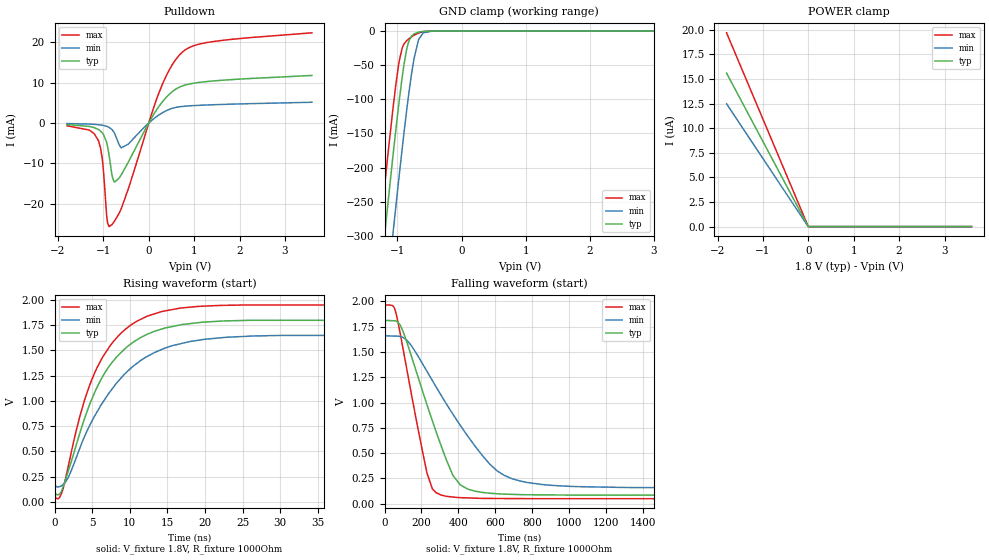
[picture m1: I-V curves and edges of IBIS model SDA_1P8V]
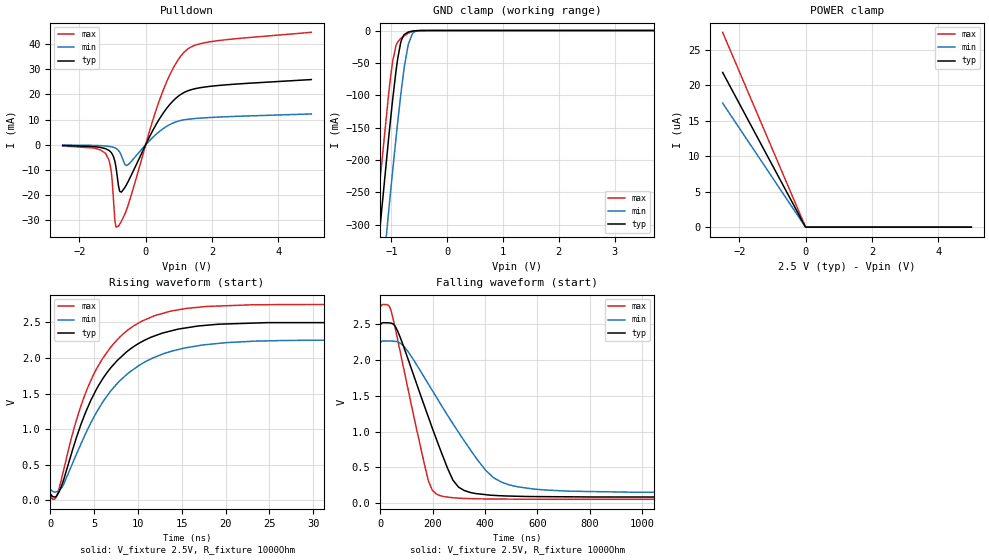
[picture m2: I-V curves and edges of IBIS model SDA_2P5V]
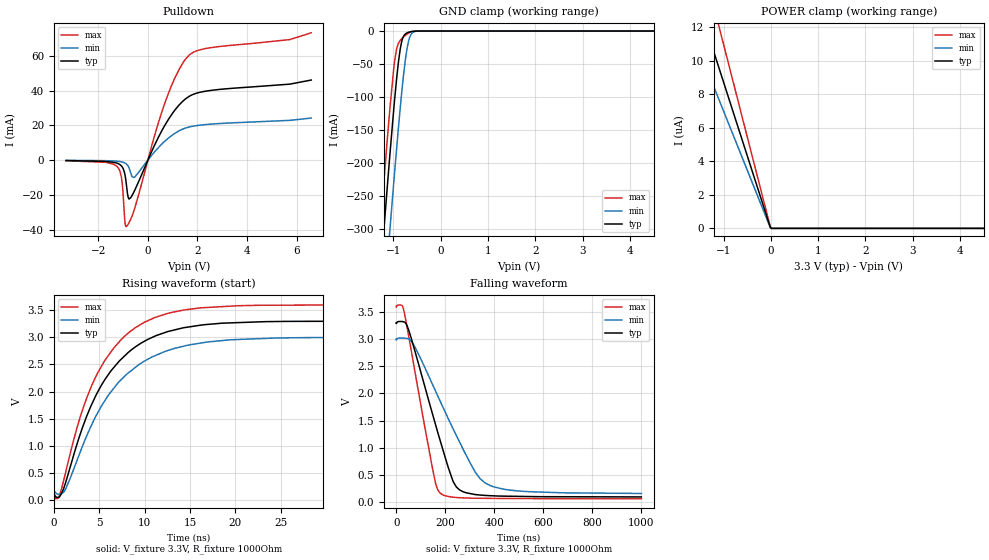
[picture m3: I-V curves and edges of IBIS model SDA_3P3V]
| Texas Instruments Incorporated
| LOW VOLTAGE 8-BIT I2C AND SMBus LOW-POWER I/O EXPANDER
| WITH INTERRUPT OUTPUT, RESET, AND CONFIGURATION REGISTERS
| Marketing part#   Voltage Range   Package-type   #pins/pkg drawing
| TCA9534PW   1.65V - 5.5V   TSSOP   16-pin PW
| TCA9534APW   1.65V - 5.5V   TSSOP   16-pin PW
[IBIS Ver]   4.1
[File name]   tca9534.ibs
[File Rev]   1.0
[Date]   09/05/2014
[Source]   Model built from spectre simulations at:
   Texas Instruments Incorporated.
   Analog-eLab, HPA
   12500 TI Blvd
   Dallas, TX -75243
   For Support e-mail: elab_ibis@list.ti.com
[Notes]   Revision History
   Rev 1.0: 09/05/2014
   - ccomp values are based on PVT settings:
   MIN: Low Voltage, High Temperature, Weak Process
   TYP: Nominal Voltage, Nominal Temperature, Nominal Process
   MAX: High Voltage, Low Temperature, Fast Process
   - C_comp although listed in numerical order of value are obtained from varying PVT conditions.
   For PVT conditions for each specific value, refer to the buffer description under respective [Model].
   IBIS model user is responsible for using appropriate C_comp to simulate for Signal Integrity.
   - Pullup and Pulldown non-monotonic for SDA, PPORT and INTZ
[Disclaimer]  This model is designed as an aid for customers of Texas Instruments
 TI and its licensors and suppliers make no warranties, either expressed
 or implied, with respect to this  model, including the warranties of
 merchantability or fitness for a particular purpose.
 The model is provided solely on an "as is" basis. The entire risk as to
 its quality and performance is with the customer.
[Copyright] (C)Copyright 2014 Texas Instruments Incorporated.
   All rights reserved.
[Component]   TCA9534PW
[Manufacturer]  Texas Instruments Incorporated
[Package]   |16-pin TSSOP PW package
|   typ   min   max
R_pkg   0.0904   0.0851   0.0990
L_pkg   3.1602n   2.6948n   3.7199n
C_pkg   0.4718p   0.4138p   0.5387p
[Pin]   signal_name   model_name   R_pin   L_pin   C_pin
1   A0   A0   0.08654  3.71131n  0.52246p
2   A1   RSTZ   0.09589  3.33166n  0.53604p
3   A2   RSTZ   0.09323  2.87657n  0.41375p
4   P0   PPORT   0.08510  2.69476n  0.41473p
5   P1   PPORT   0.08519  2.69849n  0.41486p
6   P2   PPORT   0.09338  2.88501n  0.41575p
7   P3   PPORT   0.09895  3.40069n  0.53867p
8   GND   GND   0.08515  3.68823n  0.51880p
9   P4   PPORT   0.08660  3.71993n  0.52234p
10   P5   PPORT   0.09553  3.32499n  0.53378p
11   P6   PPORT   0.09371  2.89211n  0.41437p
12   P7   PPORT   0.08555  2.70649n  0.41531p
13   INTZ   INTZ   0.08550  2.70336n  0.41534p
14   SCL   SCL   0.09363  2.88557n  0.41420p
15   SDA   SDA   0.09594  3.33276n  0.53604p
16   VCC   POWER   0.08652  3.71071n  0.52243p
[Model Selector] A0
A0_5V   A0 5V INPUT
A0_3P3V   A0 5V INPUT
A0_2P5V   A0 5V INPUT
A0_1P8V   A0 5V INPUT
[Model Selector] RSTZ
RSTZ_5V   RSTZ 5V INPUT
RSTZ_3P3V   RSTZ 5V INPUT
RSTZ_2P5V   RSTZ 5V INPUT
RSTZ_1P8V   RSTZ 5V INPUT
[Model Selector] SCL
SCL_5V   SCL 5V INPUT
SCL_3P3V   SCL 5V INPUT
SCL_2P5V   SCL 5V INPUT
SCL_1P8V   SCL 5V INPUT
[Model Selector] SDA
SDA_5V   SDA 5V INPUT
SDA_3P3V   SDA 5V INPUT
SDA_2P5V   SDA 5V INPUT
SDA_1P8V   SDA 5V INPUT
[Model Selector] INTZ
INTZ_5V   INTZ 5V INPUT
INTZ_3P3V   INTZ 5V INPUT
INTZ_2P5V   INTZ 5V INPUT
INTZ_1P8V   INTZ 5V INPUT
[Model Selector] PPORT
PPORT_5V   PPORT 5V INPUT
PPORT_3P3V   PPORT 5V INPUT
PPORT_2P5V   PPORT 5V INPUT
PPORT_1P8V   PPORT 5V INPUT
| Models and submodels in the file (24): SDA_1P8V (I/O_open_drain), SDA_2P5V (I/O_open_drain), SDA_3P3V (I/O_open_drain), SDA_5V (I/O_open_drain), PPORT_1P8V (I/O), PPORT_2P5V (I/O), PPORT_3P3V (I/O), PPORT_5V (I/O), INTZ_1P8V (Open_drain), INTZ_2P5V (Open_drain), INTZ_3P3V (Open_drain), INTZ_5V (Open_drain), SCL_1P8V (Input), SCL_2P5V (Input), SCL_3P3V (Input), SCL_5V (Input), A0_1P8V (Input), A0_2P5V (Input), A0_3P3V (Input), A0_5V (Input), RSTZ_1P8V (Input), RSTZ_2P5V (Input), RSTZ_3P3V (Input), RSTZ_5V (Input)
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|   typ   min   max
|   (nom PVT)   (fast PVT)   (slow PVT)
| Where   nom PVT is  Nominal Process, 3.3V, 27C
|   Fast PVT is Strong Process, 3.6V, -40C
|   Slow PVT is Weak Process, 3.0V, 125C
|   Model SDA_1P8V
[Model]   SDA_1P8V
Model_type   I/O_open_drain
Polarity   Non-Inverting
Enable   Active-Low
Vinl = 0.495
Vinh = 1.365
Vmeas = 0.9
Vref = 1.8
Cref = 15pF
Rref = 1000
|   typ   min   max
|   (nom PVT)   (slow PVT)   (fast PVT)
C_comp   1.545p   1.521p   1.613p
|C_comp (ON state)   1.583p   1.568p   1.703p
|C_comp (OFF state)   1.545p   1.521p   1.613p
[Voltage Range]   1.8   1.65   1.95
[Temperature Range]   27   125   -40
[Pullup Reference]   1.8   1.65   1.95
[Pulldown Reference]   -0   -0   -0
[Power Clamp Reference]   1.8   1.65   1.95
[GND Clamp Reference]   -0   -0   -0
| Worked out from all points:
|   slope of the pulldown table from 0 to 0.27 V, typ, clamps not added: 56.2 ohm
|   GND clamp passes 1 mA (typ) near -0.63 V on its own axis
|   falling waveform, V_fixture 1.8V, R_fixture 1000Ohm: 20-80 % time 191ns typ, 324ns min, 119ns max; typ from 1.8 V to 0.085 V
|   rising waveform, V_fixture 1.8V, R_fixture 1000Ohm: 20-80 % time 6.22ns typ, 7.63ns min, 5.6ns max; typ from 0.085 V to 1.8 V
[Pulldown]
|   Voltage   I(typ)   I(min)   I(max)
-1.8V     -366.8uA   -119.8uA   -673.5uA
-1.114V   -1.558mA   -398.8uA   -4.205mA
-1.028V   -2.362mA   -527.5uA   -8.5mA
-925.2mV  -4.904mA   -809.6uA   -23.01mA
-871.2mV  -8.153mA   -1.079mA   -25.67mA
-768.6mV  -14.45mA   -2.217mA   -24.55mA
-655.2mV  -13.71mA   -5.27mA    -22.42mA
-450mV    -9.681mA   -5.219mA   -16.33mA
214.2mV   3.957mA    1.938mA    7.173mA
684mV     8.95mA     4.052mA    16.97mA
1.289V    10.3mA     4.49mA     19.98mA
3.595V    11.8mA     5.162mA    22.38mA
[GND Clamp]
|   Voltage   I(typ)   I(min)   I(max)
-1.8V     -871.5mA   -985.9mA   -800.3mA
-1.444V   -528.4mA   -644.3mA   -455.8mA
-1.228V   -325.4mA   -441.4mA   -252.8mA
-1.184V   -285.7mA   -401.5mA   -213.4mA
-1.076V   -189mA     -303.3mA   -119.3mA
-984.6mV  -111.9mA   -222.4mA   -51.58mA
-925.2mV  -67.37mA   -172.1mA   -25.04mA
-844.2mV  -22.4mA    -107.8mA   -13.2mA
-741.6mV  -4.176mA   -40.63mA   -6.209mA
-666mV    -1.556mA   -11.82mA   -2.717mA
-450mV    -34.82uA   -81.17uA   -42.22uA
3.595V    0A         0A         0A
[POWER Clamp]
|   Voltage   I(typ)   I(min)   I(max)
-1.8V     15.6uA     12.48uA    19.68uA
-7.2mV    41.81nA    29.84nA    59.33nA
9mV       0A         0A         0A
3.595V    0A         0A         0A
[Ramp]
R_load = 1000
|   typ   min   max
dV/dt_r   1.02922/6.19026e-09   0.895619/7.61983e-09   1.13981/5.59782e-09
dV/dt_f   1.02922/1.90744e-07   0.895521/3.23729e-07   1.13981/1.19095e-07
[Falling Waveform]
V_fixture = 1.8V
V_fixture_min = 1.65V
V_fixture_max = 1.95V
R_fixture = 1000Ohm
C_fixture = 0F
|   Time   V(typ)   V(min)   V(max)
0s        1.8V       1.65V      1.95V
61.29ns   1.805V     1.657V     1.888V
101ns     1.698V     1.643V     1.522V
230.3ns   976.6mV    1.307V     301mV
279.4ns   711.5mV    1.154V     109.3mV
370ns     281.5mV    886.4mV    66.96mV
410ns     186.9mV    775.8mV    60.6mV
569.9ns   104.4mV    392mV      52.65mV
689.9ns   93.08mV    248.6mV    51.6mV
2us       84.64mV    157.5mV    50.32mV
[Rising Waveform]
V_fixture = 1.8V
V_fixture_min = 1.65V
V_fixture_max = 1.95V
R_fixture = 1000Ohm
C_fixture = 0F
|   Time   V(typ)   V(min)   V(max)
0s        84.63mV    157.3mV    50.31mV
483.4ps   70.29mV    147.5mV    30.62mV
1.088ns   142.6mV    171.2mV    125.1mV
3.353ns   683.8mV    534.3mV    850.8mV
4.599ns   956.5mV    748.5mV    1.147V
6.294ns   1.23V      973.7mV    1.423V
8.507ns   1.455V     1.2V       1.647V
14.95ns   1.725V     1.53V      1.895V
25.05ns   1.796V     1.637V     1.949V
2us       1.8V       1.65V      1.95V
[Model]   SDA_2P5V
Model_type   I/O_open_drain
Polarity   Non-Inverting
Enable   Active-Low
Vinl = .8
Vinh = 2
Vmeas = 1.25
Vref = 2.5
Cref = 15pF
Rref = 1000
|   typ   min   max
|   (nom PVT)   (slow PVT)   (fast PVT)
C_comp   1.492p   1.444p   1.603p
|C_comp (ON state)   1.571p   1.501p   1.693p
|C_comp (OFF state)   1.492p   1.444p   1.606p
| Where   nom PVT is  Nominal Process, 2.5V, 27C
|   Fast PVT is Strong Process, 2.75V, -40C
|   Slow PVT is Weak Process, 2.25V, 125C
[Voltage Range]   2.5   2.25   2.75
[Temperature Range]   27   125   -40
[Pullup Reference]   2.5   2.25   2.75
[Pulldown Reference]   -0   -0   -0
[Power Clamp Reference]   2.5   2.25   2.75
[GND Clamp Reference]   -0   -0   -0
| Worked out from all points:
|   slope of the pulldown table from 0 to 0.375 V, typ, clamps not added: 39.9 ohm
|   GND clamp passes 1 mA (typ) near -0.63 V on its own axis
|   falling waveform, V_fixture 2.5V, R_fixture 1000Ohm: 20-80 % time 143ns typ, 223ns min, 95.1ns max; typ from 2.5 V to 0.086 V
|   rising waveform, V_fixture 2.5V, R_fixture 1000Ohm: 20-80 % time 5.9ns typ, 6.67ns min, 5.45ns max; typ from 0.086 V to 2.5 V
[Pulldown]
|   Voltage   I(typ)   I(min)   I(max)
-2.5V     -289.2uA   -109uA     -480.5uA
-1.202V   -1.6mA     -499.8uA   -3.591mA
-1.038V   -3.122mA   -792.8uA   -10.65mA
-932.5mV  -6.351mA   -1.194mA   -29.14mA
-887.5mV  -9.521mA   -1.488mA   -32.72mA
-790mV    -18.12mA   -2.74mA    -31.69mA
-730mV    -18.79mA   -4.372mA   -30.33mA
-520mV    -14.4mA    -7.828mA   -23.65mA
425mV     10.47mA    5.375mA    18.01mA
1.16V     20.78mA    9.903mA    36.78mA
2V        23.28mA    10.86mA    41.01mA
4.992V    25.89mA    12.23mA    44.64mA
[GND Clamp]
|   Voltage   I(typ)   I(min)   I(max)
-2.5V     -1.556A    -1.668A    -1.488A
-1.472V   -555.9mA   -671.7mA   -483.5mA
-1.27V    -364.7mA   -480.8mA   -292mA
-1.21V    -309.2mA   -425.1mA   -236.7mA
-1.052V   -168.3mA   -282mA     -99.98mA
-977.5mV  -106.3mA   -216.3mA   -47.4mA
-917.5mV  -62.11mA   -165.7mA   -23.06mA
-835mV    -19.11mA   -100.9mA   -12.44mA
-700mV    -2.431mA   -21.99mA   -4.098mA
-617.5mV  -766.3uA   -4.191mA   -1.319mA
-482.5mV  -66.51uA   -170.4uA   -86.11uA
4.992V    0A         0A         0A
[POWER Clamp]
|   Voltage   I(typ)   I(min)   I(max)
-2.5V     21.83uA    17.51uA    27.48uA
-10mV     59.16nA    42.3nA     83.4nA
12.5mV    0A         0A         0A
4.992V    0A         0A         0A
[Ramp]
R_load = 1000
|   typ   min   max
dV/dt_r   1.44865/5.87927e-09   1.26147/6.64385e-09   1.6174/5.45698e-09
dV/dt_f   1.44864/1.4283e-07   1.26122/2.23363e-07   1.6174/9.51149e-08
[Falling Waveform]
V_fixture = 2.5V
V_fixture_min = 2.25V
V_fixture_max = 2.75V
R_fixture = 1000Ohm
C_fixture = 0F
|   Time   V(typ)   V(min)   V(max)
0s        2.5V       2.25V      2.75V
42.43ns   2.51V      2.262V     2.668V
90.96ns   2.166V     2.185V     1.853V
172.5ns   1.316V     1.729V     481.5mV
198.6ns   1.048V     1.573V     181.1mV
213ns     906.3mV    1.486V     131.2mV
299ns     224.6mV    988.7mV    70.75mV
402.2ns   119.6mV    459.8mV    59.59mV
492.2ns   100mV      256.4mV    57.41mV
1.5us     85.6mV     148mV      54.34mV
[Rising Waveform]
V_fixture = 2.5V
V_fixture_min = 2.25V
V_fixture_max = 2.75V
R_fixture = 1000Ohm
C_fixture = 0F
|   Time   V(typ)   V(min)   V(max)
0s        85.58mV    147.5mV    54.34mV
819.4ps   80.71mV    129mV      92.98mV
1.516ns   288.4mV    223.5mV    423mV
2.853ns   832.1mV    612.2mV    1.074V
4.287ns   1.31V      1.004V     1.589V
6.049ns   1.721V     1.394V     2.006V
7.951ns   2V         1.683V     2.296V
13.98ns   2.386V     2.1V       2.663V
22.81ns   2.488V     2.233V     2.745V
1.5us     2.5V       2.25V      2.75V
[Model]   SDA_3P3V
Model_type   I/O_open_drain
Polarity   Non-Inverting
Enable   Active-Low
Vinl = .8
Vinh = 2
Vmeas = 1.65
Vref = 3.3
Cref = 15pF
Rref = 1000
|   typ   min   max
|   typ   min   max
|   (nom PVT)   (slow PVT)   (fast PVT)
C_comp   1.485p   1.455p   1.603p
|C_comp (ON state)   1.561p   1.507p   1.688p
|C_comp (OFF state)   1.485p   1.455p   1.603p
| Where   nom PVT is  Nominal Process, 3.3V, 27C
|   Fast PVT is Strong Process, 3.6V, -40C
|   Slow PVT is Weak Process, 3.0V, 125C
[Voltage Range]   3.3   3   3.6
[Temperature Range]   27   125   -40
[Pullup Reference]   3.3   3   3.6
[Pulldown Reference]   -0   -0   -0
[Power Clamp Reference]   3.3   3   3.6
[GND Clamp Reference]   -0   -0   -0
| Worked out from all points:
|   slope of the pulldown table from 0 to 0.495 V, typ, clamps not added: 32.9 ohm
|   GND clamp passes 1 mA (typ) near -0.63 V on its own axis
|   falling waveform, V_fixture 3.3V, R_fixture 1000Ohm: 20-80 % time 122ns typ, 180ns min, 84.6ns max; typ from 3.3 V to 0.094 V
|   rising waveform, V_fixture 3.3V, R_fixture 1000Ohm: 20-80 % time 5.78ns typ, 6.32ns min, 5.39ns max; typ from 0.094 V to 3.3 V
[Pulldown]
|   Voltage   I(typ)   I(min)   I(max)
-3.3V     -240.3uA   -104.9uA   -373.7uA
-1.231V   -1.835mA   -652.4uA   -3.854mA
-1.053V   -3.586mA   -1.034mA   -11.29mA
-924mV    -8.448mA   -1.675mA   -35.67mA
-884.4mV  -12.06mA   -2.027mA   -38.17mA
-795.3mV  -21.35mA   -3.471mA   -36.81mA
-686.4mV  -21.46mA   -7.645mA   -33.71mA
-528mV    -17.21mA   -9.657mA   -27.53mA
699.6mV   20.37mA    11.09mA    33.38mA
1.254V    31.59mA    16.8mA     51.96mA
1.67V     36.68mA    19.06mA    60.37mA
6.59V     46.02mA    24.18mA    73.15mA
[GND Clamp]
|   Voltage   I(typ)   I(min)   I(max)
-3.3V     -2.346A    -2.454A    -2.279A
-1.32V    -411.5mA   -527.6mA   -338.7mA
-1.27V    -365.2mA   -481.3mA   -292.4mA
-1.201V   -301.1mA   -417mA     -228.6mA
-1.073V   -185.6mA   -299.8mA   -116.1mA
-973.5mV  -103.2mA   -212.9mA   -45.16mA
-854.7mV  -26.67mA   -115.7mA   -14.11mA
-765.6mV  -5.873mA   -54.1mA    -7.616mA
-696.3mV  -2.318mA   -20.66mA   -3.932mA
-617.1mV  -761.4uA   -4.153mA   -1.31mA
-478.5mV  -61.43uA   -155.2uA   -78.89uA
6.59V     0A         0A         0A
[POWER Clamp]
|   Voltage   I(typ)   I(min)   I(max)
-3.3V     28.92uA    23.24uA    36.36uA
-1.924V   16.82uA    13.51uA    21.16uA
-1.577V   13.79uA    11.07uA    17.35uA
-1.478V   12.92uA    10.37uA    16.26uA
-1.211V   10.58uA    8.49uA     13.31uA
-825mV    7.193uA    5.772uA    9.056uA
-13.2mV   79nA       56.82nA    110.9nA
6.6mV     0A         0A         36.96nA
16.5mV    0A         0A         0A
6.59V     0A         0A         0A
[Ramp]
R_load = 1000
|   typ   min   max
dV/dt_r   1.92356/5.75384e-09   1.70688/6.28541e-09   2.123/5.37416e-09
dV/dt_f   1.92337/1.21852e-07   1.70529/1.79636e-07   2.12298/8.45322e-08
[Falling Waveform]
V_fixture = 3.3V
V_fixture_min = 3V
V_fixture_max = 3.6V
R_fixture = 1000Ohm
C_fixture = 0F
|   Time   V(typ)   V(min)   V(max)
0s        3.3V       3V         3.6V
22.67ns   3.321V     3.017V     3.62V
32.89ns   3.313V     3.016V     3.488V
69.3ns    2.888V     2.906V     2.582V
146.2ns   1.65V      2.183V     661.9mV
177.8ns   1.154V     1.87V      170.3mV
245.4ns   276.7mV    1.221V     83.93mV
322.1ns   138.4mV    553.1mV    70mV
382.1ns   117.5mV    306mV      67.54mV
999.9ns   94.38mV    157.9mV    61.69mV
[Rising Waveform]
V_fixture = 3.3V
V_fixture_min = 3V
V_fixture_max = 3.6V
R_fixture = 1000Ohm
C_fixture = 0F
|   Time   V(typ)   V(min)   V(max)
0s        94.06mV    155.2mV    61.66mV
543.3ps   46.85mV    98.16mV    53.35mV
1.161ns   245.9mV    158.3mV    410.8mV
2.889ns   1.203V     874.5mV    1.52V
4.191ns   1.768V     1.394V     2.117V
5.625ns   2.221V     1.832V     2.574V
7.462ns   2.603V     2.226V     2.967V
12.28ns   3.092V     2.743V     3.429V
20.36ns   3.274V     2.962V     3.586V
999.9ns   3.3V       3V         3.6V
